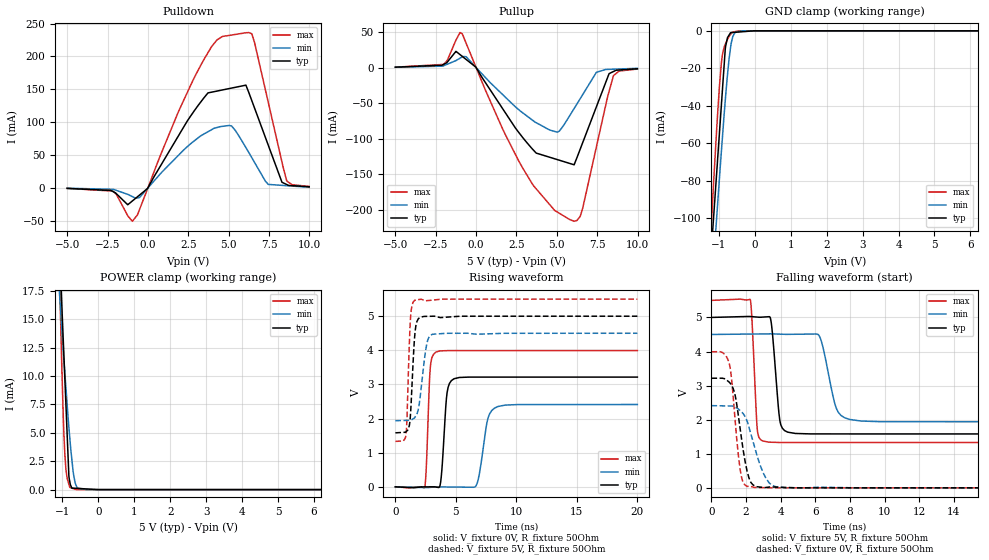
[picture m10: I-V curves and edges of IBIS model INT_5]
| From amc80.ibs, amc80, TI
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[Model]  INT_5
Model_type   3-state
Polarity   Non-Inverting
Vmeas = 2.5
Vref = 2.5
Cref = 15pF
Rref = 50
|   typ   min   max
|   (nom PVT)   (Fast PVT)   (slow PVT)
|   BUFFER OUTPUT HIGH
C_comp   1.092E-12   1.092E-12   1.164E-12
|   BUFFER OUTPUT LOW
|C_comp   1.236E-12   1.214E-12   1.271E-12
|   BUFFER HIGH Z STATE
|C_comp   1.563E-12   1.318E-12   1.828E-12
| Where   nom PVT is  Nominal Process, 5.0V, 27C
|   Fast PVT is Strong Process, 5.5V, -40C
|   Slow PVT is Weak Process, 4.5V, 125C
|C_comp - from L-C Tank method, L = 1nH, peak frequency
[Voltage Range]   5   4.5   5.5
[Temperature Range]   27   125   -40
[Pullup Reference]   5   4.5   5.5
[Pulldown Reference]   0   0   0
[Power Clamp Reference]   5   4.5   5.5
[GND Clamp Reference]   0   0   0
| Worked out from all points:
|   slope of the pulldown table from 0 to 0.75 V, typ, clamps not added: 23.2 ohm
|   slope of the pullup table from 0 to 0.75 V, typ, clamps not added: 27.6 ohm
|   GND clamp passes 1 mA (typ) near -0.67 V on its own axis
|   POWER clamp passes 1 mA (typ) near -0.81 V on its own axis
|   falling waveform, V_fixture 5V, R_fixture 50Ohm: 20-80 % time 324ps typ, 639ps min, 225ps max; typ from 5 V to 1.58 V
|   rising waveform, V_fixture 0V, R_fixture 50Ohm: 20-80 % time 344ps typ, 610ps min, 248ps max; typ from 0 V to 3.22 V
|   rising waveform, V_fixture 5V, R_fixture 50Ohm: 20-80 % time 301ps typ, 516ps min, 236ps max; typ from 1.58 V to 5 V
|   falling waveform, V_fixture 0V, R_fixture 50Ohm: 20-80 % time 573ps typ, 875ps min, 429ps max; typ from 3.22 V to 0 V
[Pulldown]
|   Voltage   I(typ)   I(min)   I(max)
-5V       -736.2uA   -519.2uA   -724.3uA
-2.168V   -5.495mA   -2.14mA    -4.899mA
-961.3mV  -19.84mA   -13.29mA   -50.82mA
-17.11mV  -777.9uA   -492uA     -1.087mA
1.969V    82.45mA    51.58mA    120.2mA
3.925V    145.6mA    88.31mA    214.1mA
5.182V    151.9mA    94.19mA    232.6mA
6.243V    145.4mA    54.05mA    236.3mA
6.601V    121.7mA    38.87mA    221.5mA
7.455V    64.84mA    5.311mA    130mA
8.59V     5.195mA    3.361mA    11.19mA
9.985V    1.703mA    965.1uA    2.2mA
[GND Clamp]
|   Voltage   I(typ)   I(min)   I(max)
-5V       -1.381A    -1.29A     -1.545A
-1.238V   -126.6mA   -151.3mA   -115.4mA
-1.136V   -98.09mA   -122.2mA   -79.26mA
-1.084V   -83.83mA   -107.6mA   -62.15mA
-1.047V   -73.42mA   -97.34mA   -49.66mA
-918.7mV  -37.96mA   -62.91mA   -16.2mA
-816.3mV  -9.574mA   -37.1mA    -7.228mA
-755.6mV  -3.678mA   -23.66mA   -4.617mA
-669.1mV  -994uA     -8.907mA   -1.933mA
-545.5mV  -805.5uA   -853.3uA   -438.3uA
-347.5mV  -503.7uA   -4.497uA   -2.812uA
9.985V    0A         0A         0A
[Pullup]
|   Voltage   I(typ)   I(min)   I(max)
-5V       581.8uA    454.9uA    619.1uA
-2.011V   4.527mA    2.646mA    4.591mA
-1.25V    22.88mA    9.852mA    38.7mA
-870.5mV  16.05mA    15.01mA    47.98mA
-17.11mV  657.7uA    429uA      952.3uA
2.867V    -98mA      -63.39mA   -140.8mA
5.032V    -129.7mA   -90.98mA   -203.6mA
6.066V    -136.9mA   -57.8mA    -216.6mA
6.597V    -105.9mA   -38.19mA   -198.4mA
7.455V    -54.87mA   -6.563mA   -111.1mA
8.511V    -5.455mA   -2.231mA   -11.23mA
9.985V    -1.656mA   -1.033mA   -2.065mA
[POWER Clamp]
|   Voltage   I(typ)   I(min)   I(max)
-5V       454mA      315.5mA    657.3mA
-1.067V   20.42mA    16.77mA    17.67mA
-1.058V   19.73mA    16.34mA    16.47mA
-1.016V   16.48mA    14.32mA    11.13mA
-970.5mV  13.02mA    12.17mA    6.279mA
-928.9mV  9.829mA    10.3mA     3.134mA
-894.4mV  7.185mA    8.803mA    1.678mA
-816.3mV  1.2mA      5.498mA    475.2uA
-783.7mV  569.3uA    4.285mA    184.3uA
-641.5mV  120.3uA    570.9uA    32.55uA
-313.8mV  57.16uA    45.21nA    442.7nA
9.985V    0A         0A         0A
[Ramp]
R_load = 50
|   typ   min   max
dV/dt_r   1.92936/3.42406e-010   1.44734/6.02752e-010   2.39556/2.47048e-010
dV/dt_f   2.05119/3.21585e-010   1.53749/6.32684e-010   2.50192/2.24456e-010
[Falling Waveform]
V_fixture = 5V
V_fixture_min = 4.5V
V_fixture_max = 5.5V
R_fixture = 50Ohm
C_fixture = 0F
|   Time   V(typ)   V(min)   V(max)
0s        5V         4.5V       5.5V
2.242ns   5.027V     4.512V     5.521V
2.642ns   5.011V     4.514V     1.731V
2.959ns   5.01V      4.516V     1.376V
3.405ns   4.976V     4.519V     1.339V
3.942ns   2.002V     4.51V      1.331V
4.401ns   1.635V     4.504V     1.331V
6.21ns    1.583V     4.471V     1.331V
7.967ns   1.582V     2.009V     1.331V
20ns      1.581V     1.938V     1.33V
[Rising Waveform]
V_fixture = 0V
V_fixture_min = 0V
V_fixture_max = 0V
R_fixture = 50Ohm
C_fixture = 0F
|   Time   V(typ)   V(min)   V(max)
0s        89.62nV    166.6nV    54.97nV
2.427ns   -1.666mV   -21.41mV   -8.712mV
2.878ns   -570.8uV   -16.26mV   3.459V
3.353ns   -5.697mV   -4.872mV   3.949V
3.746ns   149.4mV    -2.591mV   3.983V
4.272ns   2.752V     -4.562mV   3.991V
4.846ns   3.166V     -6.715mV   3.992V
6.68ns    3.215V     37.2mV     3.992V
8.481ns   3.215V     2.354V     3.992V
20ns      3.216V     2.412V     3.993V
[Rising Waveform]
V_fixture = 5V
V_fixture_min = 4.5V
V_fixture_max = 5.5V
R_fixture = 50Ohm
C_fixture = 0F
|   Time   V(typ)   V(min)   V(max)
0s        1.581V     1.938V     1.33V
881ps     1.612V     1.947V     1.533V
948ps     1.636V     1.947V     1.912V
1.141ns   1.779V     1.949V     4.068V
1.25ns    2.126V     1.95V      4.949V
1.609ns   4.467V     2.037V     5.469V
1.984ns   4.95V      2.452V     5.49V
2.592ns   4.995V     4.181V     5.454V
3.066ns   4.999V     4.471V     5.471V
20ns      5V         4.5V       5.5V
[Falling Waveform]
|Gnd
V_fixture = 0V
V_fixture_min = 0V
V_fixture_max = 0V
R_fixture = 50Ohm
C_fixture = 0F
|   Time   V(typ)   V(min)   V(max)
0s        3.216V     2.412V     3.993V
1.028ns   3.099V     2.402V     3.644V
1.159ns   3.011V     2.401V     3.206V
1.343ns   2.774V     2.37V      2.121V
1.645ns   1.776V     2.269V     578.1mV
2.047ns   516mV      1.971V     43.77mV
2.404ns   84.42mV    1.352V     21.6mV
2.987ns   10.43mV    440.4mV    6.666mV
3.729ns   21.6mV     33.13mV    627.1uV
20ns      89.64nV    166.6nV    54.99nV
